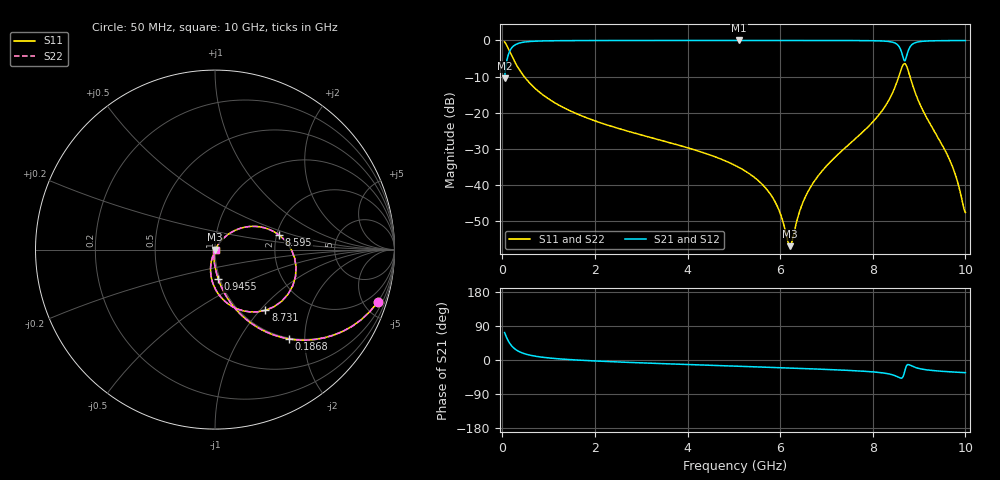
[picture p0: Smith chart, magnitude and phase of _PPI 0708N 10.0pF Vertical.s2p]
! S-Parameter data specifications (vertical orientation):
! Substrate: 40-mil Rogers 3003C, Substrate thickness, H=1.016mm, Dielectric constant, Er=3, Conductor thickness, T_mtl=0.043mm, Loss Tangent, Tand=0.003
! PCB Mounting Pad Footprint: Pad width, PadW=2.54mm , Pad length, PadL=0.51mm , Pad gap, PadG (edge-to-edge)=0.71mm , Reference planes=1.73mm apart
! Created Tue Jan 16 08:47:00 2018
# GHz S MA R 50
! 2 Port Network Data from SP1.SP block
! freq  magS11  angS11  magS21  angS21  magS12  angS12  magS22  angS22
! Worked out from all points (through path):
!   801 points, 50 MHz to 10 GHz, reference 50 ohm
!   highest |S21| = -0.01 dB at 5.112 GHz (marker M1); lowest = -10.4 dB at 50 MHz (marker M2)
!   group delay of S21, straight-line fit = 14.1 ps
!   lowest |S11| = -56.8 dB at 6.207 GHz (marker M3), VSWR 1.00, Z = 50.1 - j0.0659 ohm
!   |S11| at or under -10 dB: 473.8 MHz to 8.561 GHz (8.088 GHz wide, 179 % of centre); 8.804 GHz to end of sweep
!   |S22| runs from -56.8 to -0.4 dB; largest |S21 - S12| = 0
!   S11 on the Smith chart (normalised r, x): 50 MHz: 0.98, -6.26; 186.8 MHz: 0.98, -1.68; 945.5 MHz: 0.98, -0.33; 8.595 GHz: 2.07, +0.38; 8.731 GHz: 1.28, -1.07; 10 GHz: 1.01, -0.01
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0.05  0.9534 -17.7  0.3016 72.3  0.3016 72.3  0.9534 -17.7
0.1868125  0.6457 -50.4  0.7633 39.6  0.7633 39.6  0.6457 -50.4
0.2863125  0.4831 -62.1  0.8753 27.9  0.8753 27.9  0.4831 -62.1
0.423125  0.3497 -71.0  0.9365 19.0  0.9365 19.0  0.3497 -71.0
0.9455  0.1645 -83.7  0.9859 6.2  0.9859 6.2  0.1645 -83.7
1.716625  0.09076 -90.4  0.9952 -0.8  0.9952 -0.8  0.09076 -90.4
3.370812  0.04271 -98.1  0.9981 -9.2  0.9981 -9.2  0.04271 -98.1
5.025  0.01883 -102.8  0.9985 -16.2  0.9985 -16.2  0.01883 -102.8
5.112063  0.01761 -102.9  0.9985 -16.6  0.9985 -16.6  0.01761 -102.9
5.808562  0.007228 -99.2  0.9984 -19.5  0.9984 -19.5  0.007228 -99.2
5.995125  0.004195 -91.5  0.9984 -20.3  0.9984 -20.3  0.004195 -91.5
6.206563  0.001442 -27.1  0.9983 -21.2  0.9983 -21.2  0.001442 -27.1
6.46775  0.005306 50.5  0.9982 -22.4  0.9982 -22.4  0.005306 50.5
6.691625  0.01027 57.1  0.998 -23.4  0.998 -23.4  0.01027 57.1
8.345812  0.1491 44.5  0.9658 -36.7  0.9658 -36.7  0.1491 44.5
8.594563  0.3668 12.7  0.7657 -47.6  0.7657 -47.6  0.3668 12.7
8.669187  0.4726 -18.3  0.5429 -38.7  0.5429 -38.7  0.4726 -18.3
8.731375  0.4395 -50.3  0.6095 -14.5  0.6095 -14.5  0.4395 -50.3
8.818437  0.2939 -79.0  0.8382 -14.3  0.8382 -14.3  0.2939 -79.0
8.942813  0.1712 -95.7  0.942 -20.6  0.942 -20.6  0.1712 -95.7
9.676625  0.0212 -106.3  0.9939 -31.3  0.9939 -31.3  0.0212 -106.3
10  0.004202 -38.8  0.9954 -33.4  0.9954 -33.4  0.004202 -38.8
